(* Logix 5000 AddOnInstructionDefinition export AMCI_SD4840E2_Disable_Driver; software revision 20.03 *)

ADD_ON_INSTRUCTION AMCI_SD4840E2_Disable_Driver   (* revision 1.0, vendor AMCI *)
VAR_IN_OUT
   AMCI_SD4840E2_output_data : _000A:SD4840E2_4342D302:O:0; {required}
END_VAR
VAR
   command_data_block : INT[10];
        [0]   // Command Bits MSW
        [1]   // Command Bits LSW
        [2]   // Upper Target Position
        [3]   // Lower Target Position
        [4]   // Upper Programmed Speed
        [5]   // Lower Programmed Speed
END_VAR

ROUTINE Logic   (* ladder *)
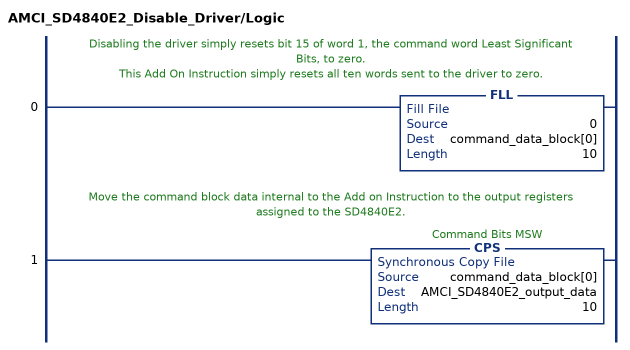
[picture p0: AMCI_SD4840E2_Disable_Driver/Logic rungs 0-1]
   // Disabling the driver simply resets bit 15 of word 1, the command word Least Significant Bits, to zero.
   // This Add On Instruction simply resets all ten words sent to the driver to zero.
   0: FLL(0,command_data_block[0],10);
   // Move the command block data internal to the Add on Instruction to the output registers assigned to the SD4840E2.
   1: CPS(command_data_block[0],AMCI_SD4840E2_output_data,10);
END_ROUTINE
END_ADD_ON_INSTRUCTION
